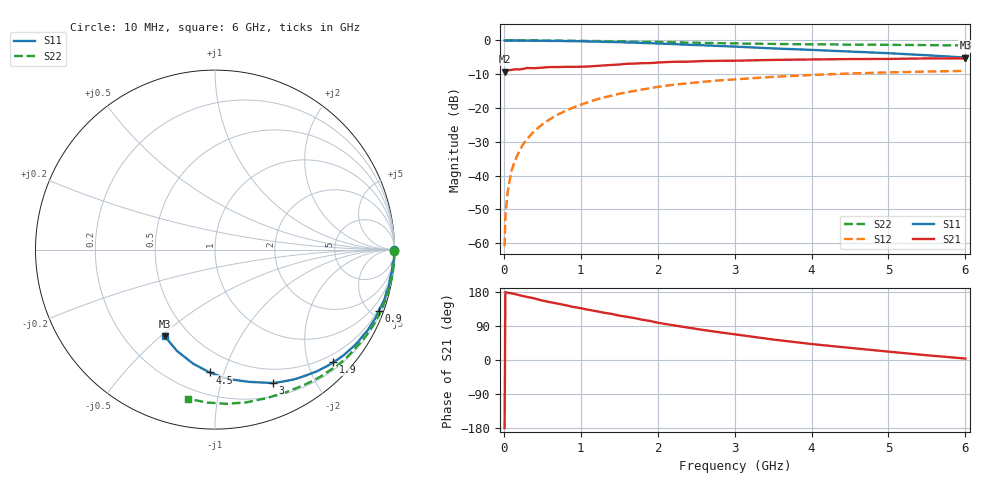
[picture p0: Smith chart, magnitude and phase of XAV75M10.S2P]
! SIEMENS Discrete & RF Semiconductors
! BFY180
! Si NPN RF Bipolar Junction Transistor in MICRO-X
! VCE = 0.75 V  IC = 0.1 mA
! Common Emitter S-Parameters:  May  1997
# GHz  S  MA  R  50
!  f  S11  S21  S12  S22
! GHz  MAG  ANG  MAG  ANG  MAG  ANG  MAG  ANG
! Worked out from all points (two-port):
!   36 points, 10 MHz to 6 GHz, reference 50 ohm
!   highest |S21| = -5.30 dB at 6 GHz (marker M1); lowest = -9.2 dB at 10 MHz (marker M2)
!   |S21| within 3 dB of the highest: 272.8 MHz to end of sweep
!   lowest |S11| = -5.1 dB at 6 GHz (marker M3), VSWR 3.53, Z = 18.4 - j25.8 ohm
!   |S11| at or under -10 dB: nowhere
!   |S22| runs from -1.5 to 0.0 dB; largest |S21 - S12| = 0.39
!   S11 on the Smith chart (normalised r, x): 10 MHz: open; 900 MHz: 0.42, -5.47; 1.9 GHz: 0.34, -2.46; 3 GHz: 0.34, -1.47; 4.5 GHz: 0.35, -0.90; 6 GHz: 0.37, -0.52
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0.01  0.9978 -0.1  0.345 -179.9  0.0009 89.7  0.9999 -0.3
0.02  0.9989 -0.3  0.365 179.1  0.0025 88.7  0.9999 -0.4
0.05  0.9949 -1.1  0.361 177.6  0.0058 89.1  0.9994 -1.0
0.1  0.9986 -2.3  0.367 175.8  0.0119 89.0  0.9997 -2.1
0.15  0.9989 -3.5  0.375 173.8  0.0171 87.4  0.9999 -3.1
0.2  0.9924 -4.4  0.372 171.0  0.0228 85.2  0.9994 -4.1
0.25  0.993 -5.8  0.379 168.7  0.0289 84.7  0.9999 -5.1
0.3  0.9937 -6.8  0.391 166.5  0.0345 83.9  0.9992 -6.0
0.4  0.9883 -9.1  0.388 162.4  0.0462 81.7  0.9984 -8.0
0.6  0.9838 -13.8  0.404 152.5  0.0684 77.4  0.9943 -12.1
0.9  0.9734 -20.6  0.407 140.2  0.1012 70.4  0.988 -18.2
1.1  0.9664 -25.1  0.412 132.6  0.1222 66.3  0.9825 -22.1
1.5  0.9436 -34.5  0.44 117.2  0.1622 57.5  0.9686 -30.0
1.9  0.9099 -43.6  0.462 103.1  0.1961 49.5  0.9516 -37.6
2.2  0.8841 -50.1  0.483 91.7  0.2202 43.5  0.9406 -43.1
2.6  0.8475 -58.5  0.496 79.0  0.2451 36.3  0.9209 -49.8
3  0.8112 -66.4  0.501 67.8  0.2652 29.2  0.9033 -56.4
3.5  0.7622 -75.3  0.515 54.1  0.2891 21.9  0.8882 -63.7
4  0.7246 -84.3  0.523 42.1  0.3079 14.5  0.8755 -71.1
4.5  0.6851 -92.5  0.53 32.0  0.324 7.6  0.8689 -78.4
5.5  0.6039 -110.4  0.542 12.5  0.3461 -5.9  0.8531 -93.2
6  0.5583 -120.2  0.543 3.8  0.3543 -12.7  0.8442 -100.4
